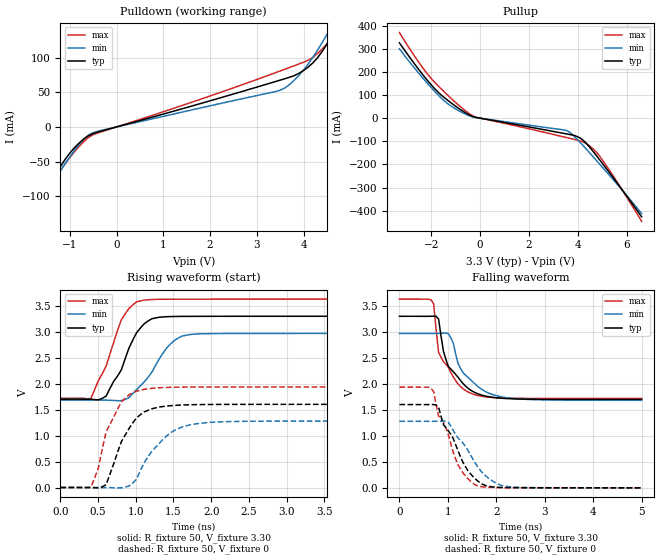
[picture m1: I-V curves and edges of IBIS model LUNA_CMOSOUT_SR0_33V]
[IBIS Ver]   3.2
[Comment Char]   |_char
[File name]   sg8201cga_33v_e.ibs
[File Rev]   1.1
[Date]   2021/10/19 9:35:58
[Source]
[Notes]
[Disclaimer]
This information is for modeling purposes only, and is not guaranteed.
Property of SEIKO EPSON Corp.,
unauthorized reproduction and/or distribution is strictly prohibited.
[Copyright]
Copyright 2021, SEIKO EPSON Corp.
[Component]   2G005_2016
Si_location Pin
Timing_location Pin
[Manufacturer]   SEIKO EPSON Corp.
| 2016 PKG
[Package]
R_pkg   42m   NA   NA
L_pkg   0.49n   NA   NA
C_pkg   0.178p   NA   NA
[Pin] signal_name   model_name
1   OE   NC
2   GND   GND
3   OUT   LUNA_CMOSOUT_SR0_33V
4   VCC   POWER
| Models and submodels in the file (1): LUNA_CMOSOUT_SR0_33V (Output)
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[Model]   LUNA_CMOSOUT_SR0_33V
Model_type Output
Polarity Non-Inverting
Vmeas=1.65
C_comp   2.5p   2.0p   3.0p
[Temperature Range] 25   140   -40
[Voltage Range]   3.30   2.97   3.63
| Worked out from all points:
|   slope of the pulldown table from 0 to 0.495 V, typ, clamps not added: 54.3 ohm
|   slope of the pullup table from 0 to 0.495 V, typ, clamps not added: 53.8 ohm
|   falling waveform, R_fixture 50, V_fixture 3.30: 20-80 % time 449ps typ, 503ps min, 397ps max; typ from 3.3 V to 1.7 V
|   falling waveform, R_fixture 50, V_fixture 0: 20-80 % time 535ps typ, 587ps min, 476ps max; typ from 1.6 V to 0.001 V
|   rising waveform, R_fixture 50, V_fixture 3.30: 20-80 % time 312ps typ, 377ps min, 294ps max; typ from 1.7 V to 3.3 V
|   rising waveform, R_fixture 50, V_fixture 0: 20-80 % time 306ps typ, 397ps min, 267ps max; typ from 0 V to 1.6 V
[Pullup]
-3.3V     325.7mA    299.8mA    370.1mA
-2.4V     195.3mA    180.3mA    225.5mA
-1.8V     121mA      109.1mA    148.7mA
-1.2V     67.06mA    53.18mA    86.77mA
-300mV    6.942mA    5.417mA    9.797mA
3.5V      -67.42mA   -52.76mA   -83.19mA
3.7V      -71.4mA    -64.51mA   -88.3mA
4.1V      -86.9mA    -106.3mA   -98.75mA
4.5V      -128.6mA   -153mA     -122.6mA
4.8V      -168.4mA   -188.7mA   -153.1mA
5.1V      -209.8mA   -224.8mA   -196.4mA
6.6V      -426.3mA   -412.6mA   -445.9mA
[Pulldown]
-3.3V     -314.8mA   -297.7mA   -349.1mA
-2V       -149.9mA   -147.7mA   -162.1mA
-1.9V     -137.8mA   -136.9mA   -148.4mA
-1.1V     -46.93mA   -53mA      -53.53mA
-700mV    -17.46mA   -17.36mA   -21.24mA
-500mV    -9.507mA   -8.246mA   -11.16mA
3.6V      69.61mA    56.27mA    83.31mA
4.2V      92.4mA     100.5mA    100.4mA
4.6V      130.8mA    145.2mA    127.5mA
4.7V      143.2mA    157.3mA    136mA
4.8V      156.3mA    169.6mA    145.3mA
6.6V      438.4mA    415.9mA    455.8mA
[Falling Waveform]
R_fixture=50
V_fixture=3.30
V_fixture_min=2.97
V_fixture_max=3.63
0s        3.3V       2.97V      3.63V
656.6ps   3.301V     2.97V      3.615V
707.1ps   3.302V     2.97V      3.536V
808.1ps   3.247V     2.97V      2.61V
909.1ps   2.625V     2.977V     2.428V
1.01ns    2.335V     2.964V     2.316V
1.263ns   2.063V     2.295V     1.948V
1.515ns   1.854V     2.039V     1.803V
2.323ns   1.714V     1.722V     1.724V
5ns       1.702V     1.685V     1.72V
[Falling Waveform]
R_fixture=50
V_fixture=0
V_fixture_min=0
V_fixture_max=0
0s        1.603V     1.281V     1.938V
707.1ps   1.602V     1.28V      1.851V
808.1ps   1.553V     1.281V     1.381V
909.1ps   1.216V     1.285V     1.268V
1.01ns    1.096V     1.263V     1.023V
1.212ns   708.7mV    955.8mV    439.6mV
1.414ns   331.5mV    724mV      175.8mV
1.616ns   133.1mV    402.7mV    39.12mV
2.222ns   6.32mV     26.6mV     3.305mV
5ns       624.5uV    1.004mV    394.7uV
[Rising Waveform]
R_fixture=50
V_fixture=3.30
V_fixture_min=2.97
V_fixture_max=3.63
0s        1.702V     1.685V     1.72V
404ps     1.702V     1.685V     1.713V
606.1ps   1.762V     1.684V     2.339V
808.1ps   2.267V     1.674V     3.235V
909.1ps   2.686V     1.732V     3.45V
1.01ns    2.982V     1.888V     3.578V
1.212ns   3.251V     2.22V      3.622V
1.414ns   3.292V     2.697V     3.628V
1.667ns   3.298V     2.934V     3.629V
5ns       3.3V       2.97V      3.63V
[Rising Waveform]
R_fixture=50
V_fixture=0
V_fixture_min=0
V_fixture_max=0
0s        0V         617.5nV    0V
404ps     -538.5uV   243.1uV    7.057mV
505.1ps   -6.748mV   398.6uV    383.4mV
606.1ps   56.54mV    -662.8uV   1.075V
808.1ps   882mV      -5.88mV    1.648V
959.6ps   1.244V     84.95mV    1.822V
1.061ns   1.403V     326.3mV    1.875V
1.414ns   1.57V      1.002V     1.929V
1.768ns   1.596V     1.22V      1.936V
5ns       1.603V     1.281V     1.938V
[Ramp]
R_load=50
dV/dt_r   9.615E-1/3.040E-10   7.684E-1/3.965E-10   1.163E+0/2.656E-10
dV/dt_f   9.586E-1/4.468E-10   7.709E-1/5.028E-10   1.146E+0/3.972E-10
|[End   LUNA_CMOSOUT_SR0_33V
